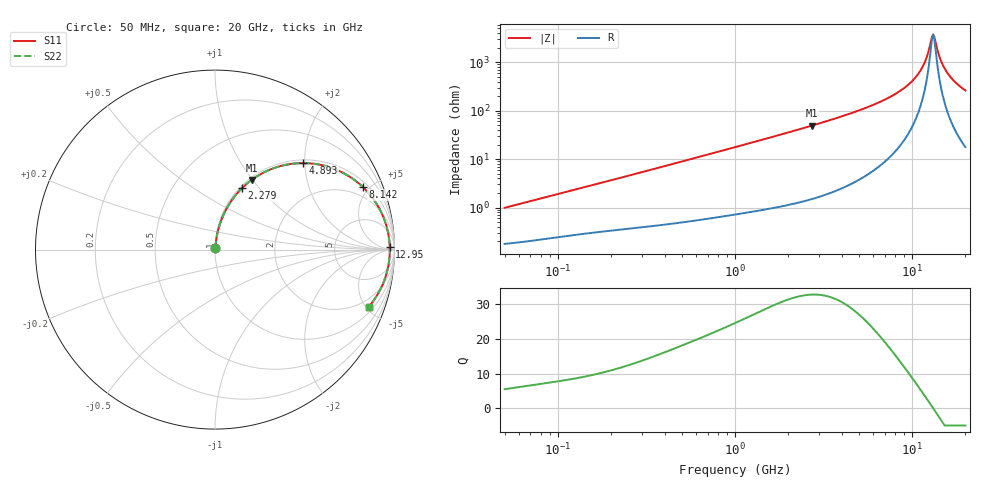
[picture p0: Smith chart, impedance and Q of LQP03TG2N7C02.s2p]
!Murata Part Number: LQP03TG2N7C02
!These Parameters are Measured in Series Mode Connection
!  o--[Z]--o
!Port1  Port2
!  o-------o
!Freq. Start=50[MHz] Stop=20[GHz], 401[Steps]
# Hz S RI R 50
!Freq.(Hz) S11(Real) S11(Imag) S21(Real) S21(Imag) S12(Real) S12(Imag) S22(Real) S22(Imag)
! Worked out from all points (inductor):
!   401 points, 50 MHz to 20 GHz, reference 50 ohm
!   read as one part in series: L = 3.07 nH near 51.52 MHz
!   highest Q = 32.8 at 2.728 GHz (marker M1), where L = 2.88 nH
!   self-resonance near 13.15 GHz
!   S11 on the Smith chart (normalised r, x): 50 MHz: 1.00, +0.02; 2.279 GHz: 1.03, +0.82; 4.893 GHz: 1.07, +1.96; 8.142 GHz: 1.30, +4.54; 12.95 GHz: 61, +30; 20 GHz: 1.35, -5.24
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5e7  0.00187 0.00971  0.9981 -0.00971  0.9981 -0.00971  0.00187 0.00971
1.364002e8  0.00347 0.0252  0.9965 -0.0252  0.9965 -0.0252  0.00347 0.0252
3.721004e8  0.00866 0.0658  0.9913 -0.0658  0.9913 -0.0658  0.00866 0.0658
1e9  0.0367 0.1687  0.9633 -0.1687  0.9633 -0.1687  0.0367 0.1687
1.567309e9  0.0787 0.2527  0.9213 -0.2527  0.9213 -0.2527  0.0787 0.2527
2.279204e9  0.1502 0.3421  0.8498 -0.3421  0.8498 -0.3421  0.1502 0.3421
2.728004e9  0.2034 0.3875  0.7966 -0.3875  0.7966 -0.3875  0.2034 0.3875
3.626126e9  0.3208 0.4513  0.6792 -0.4513  0.6792 -0.4513  0.3208 0.4513
4.89267e9  0.491 0.4821  0.509 -0.4821  0.509 -0.4821  0.491 0.4821
6.034176e9  0.6299 0.4615  0.3701 -0.4615  0.3701 -0.4615  0.6299 0.4615
7.442007e9  0.7684 0.3942  0.2316 -0.3942  0.2316 -0.3942  0.7684 0.3942
8.141811e9  0.8224 0.3501  0.1776 -0.3501  0.1776 -0.3501  0.8224 0.3501
9.745021e9  0.9109 0.2372  0.0891 -0.2372  0.0891 -0.2372  0.9109 0.2372
1.098561e10  0.9505 0.1472  0.0495 -0.1472  0.0495 -0.1472  0.9505 0.1472
1.183995e10  0.9658 0.087  0.0342 -0.087  0.0342 -0.087  0.9658 0.087
1.295331e10  0.9738 0.0125  0.0262 -0.0125  0.0262 -0.0125  0.9738 0.0125
1.314879e10  0.974 1.33e-05  0.026 -1.33e-05  0.026 -1.33e-05  0.974 1.33e-05
1.334722e10  0.9739 -0.0125  0.0261 0.0125  0.0261 0.0125  0.9739 -0.0125
1.460232e10  0.9664 -0.0871  0.0336 0.0871  0.0336 0.0871  0.9664 -0.0871
1.573793e10  0.9516 -0.1476  0.0484 0.1476  0.0484 0.1476  0.9516 -0.1476
1.747767e10  0.9184 -0.2274  0.0816 0.2274  0.0816 0.2274  0.9184 -0.2274
2e10  0.8571 -0.3177  0.1429 0.3177  0.1429 0.3177  0.8571 -0.3177
